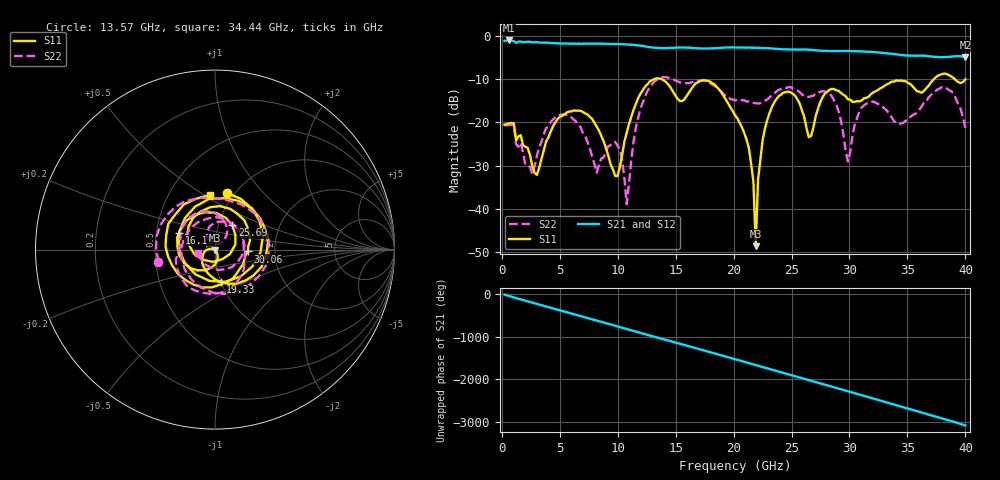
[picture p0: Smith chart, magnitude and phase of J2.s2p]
!Agilent Technologies,E8364B,MY43040528,A.07.50.67
!Agilent E8364B: A.07.50.67
!Date: Thursday, May 22, 2025 22:28:57
!Correction: S11(Full 2 Port(1,2))
!S21(Full 2 Port(1,2))
!S12(Full 2 Port(1,2))
!S22(Full 2 Port(1,2))
!S2P File: Measurements: S11, S21, S12, S22:
# Hz S  dB  R 50
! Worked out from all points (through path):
!   201 points, 250 MHz to 40 GHz, reference 50 ohm
!   highest |S21| = -1.05 dB at 647.5 MHz (marker M1); lowest = -5.0 dB at 40 GHz (marker M2)
!   group delay of S21, straight-line fit = 213 ps
!   lowest |S11| = -48.6 dB at 21.91 GHz (marker M3), VSWR 1.01, Z = 49.8 - j0.277 ohm
!   |S11| at or under -10 dB: start of sweep to 13.15 GHz; 13.79 GHz to 37.28 GHz (23.49 GHz wide, 92 % of centre); 39.08 GHz to end of sweep
!   |S22| runs from -38.9 to -9.5 dB; largest |S21 - S12| = 0.01
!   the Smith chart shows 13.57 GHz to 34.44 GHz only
!   S11 on the Smith chart (normalised r, x): 13.57 GHz: 0.93, +0.65; 16.15 GHz: 0.66, +0.13; 19.33 GHz: 1.00, -0.37; 25.69 GHz: 1.16, +0.33; 30.06 GHz: 1.45, -0.03; 34.44 GHz: 0.79, +0.53
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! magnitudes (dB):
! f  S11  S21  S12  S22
! 250 MHz  -20.6  -1.2  -1.2  -20.7
! 647.5 MHz  -20.2  -1.1  -1.0  -20.6
! 3.033 GHz  -32.2  -1.5  -1.4  -27.7
! 7.008 GHz  -17.6  -1.8  -1.8  -22.5
! 9.79 GHz  -32.4  -1.9  -1.9  -24.5
! 10.78 GHz  -22.4  -2.0  -2.0  -38.9
! 11.78 GHz  -14.3  -2.2  -2.2  -18.8
! 13.57 GHz  -9.8  -2.8  -2.8  -9.8
! 16.15 GHz  -13.1  -2.7  -2.7  -10.9
! 19.33 GHz  -14.7  -2.7  -2.7  -13.9
! 20.12 GHz  -18.3  -2.7  -2.7  -14.9
! 21.32 GHz  -25.9  -2.7  -2.7  -15.2
! 21.91 GHz  -48.6  -2.8  -2.8  -15.6
! 22.11 GHz  -33.3  -2.8  -2.8  -15.7
! 22.91 GHz  -19.4  -2.8  -2.9  -14.7
! 25.69 GHz  -15.6  -3.2  -3.1  -12.9
! 26.88 GHz  -21.2  -3.3  -3.3  -13.9
! 30.06 GHz  -14.8  -3.5  -3.5  -27.0
! 33.44 GHz  -11.0  -4.1  -4.1  -18.1
! 34.44 GHz  -10.3  -4.4  -4.4  -20.3
! 38.21 GHz  -8.7  -4.9  -4.9  -11.8
! 40 GHz  -10.0  -5.0  -4.9  -21.2
